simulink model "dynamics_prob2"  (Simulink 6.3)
settings: Solver=ode3  StartTime=start_time  StopTime=stop_time  FixedStep=time_step  RelTol=1e-3

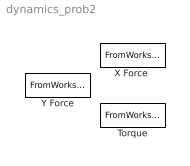
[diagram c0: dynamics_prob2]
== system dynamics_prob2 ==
  Torque : FromWorkspace  VariableName=torque  SampleTime=0.01  Interpolate=off  OutputAfterFinalValue=Holding final value
  "X Force " : FromWorkspace  VariableName=x_force  SampleTime=0.01  Interpolate=off  OutputAfterFinalValue=Holding final value
  Y Force : FromWorkspace  VariableName=y_force  SampleTime=0.01  Interpolate=off  OutputAfterFinalValue=Holding final value
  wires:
  "X Force "/1 -> ?
  Y Force/1 -> ?
  Torque/1 -> ?
